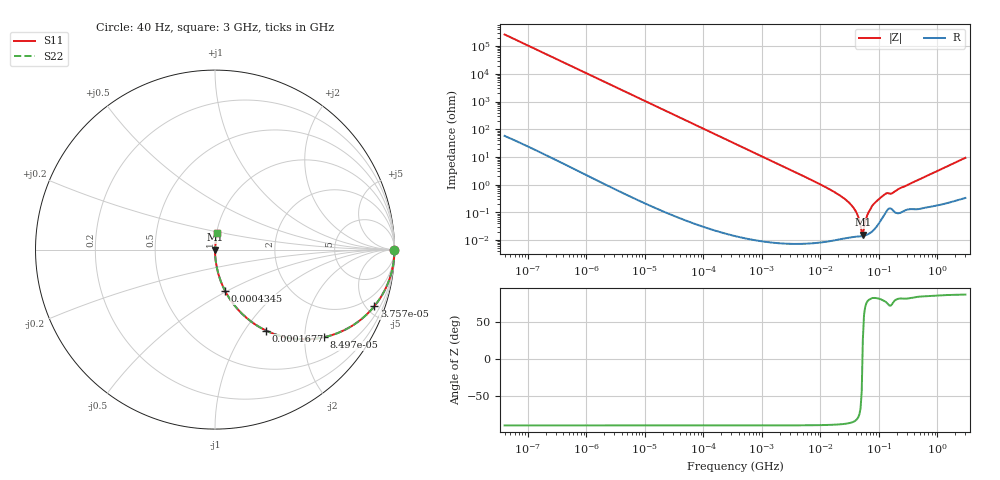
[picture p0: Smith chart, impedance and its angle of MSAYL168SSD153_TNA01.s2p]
! MSAYL168SSD153_TNA01  S-PARAMETER MODEL  ( General Type )
! Model Generated by TAIYO YUDEN Corporation (http://www.ty-top.com)
! Version 3.0
! TAIYO YUDEN Control No. 160201
! Copyright(c) 2003 TAIYO YUDEN CO.,LTD. All Rights Reserved.
! Product Description (link to TY-COMPAS)
! https://ds.yuden.co.jp/TYCOMPAS/or/detail?pn=MSAYL168SSD153KTNA01&u=M
! Products Name : Multilayer Ceramic Capacitors
! Characteristics :
!  Capacitance : 0.015 uF , Rated Voltage : 10V
!  Case Size : 1.6 x 0.8 / 0.063 x 0.031 [mm/inch] , Thickness : 0.8 / 0.031 [mm/inch]
!  (Conditions: Temperature = 25 degC , DC Bias Current/Voltage = 0A / 0V)
! External Node Assignments :
!  1  o---| |---o  2
! GND o---------o GND
! Frequency Range : 0.00004MHz  -  3000MHz  [ 401 STEP ]
# MHz S RI R 50
! Freq[MHz].  S11 Real  S11 Imag  S21 Real  S21 Imag  S12 Real  S12 Imag  S22 Real  S22 Imag
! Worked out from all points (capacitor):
!   401 points, 40 Hz to 3 GHz, reference 50 ohm
!   read as one part in series: C = 15.1 nF near 44 Hz
!   lowest |Z| = 15.8 mohm at 53.08 MHz (marker M1)
!   series resonance near 52.25 MHz, so ESL is about 620 pH
!   S11 on the Smith chart (normalised r, x): 40 Hz: open; 37.58 kHz: 1.00, -5.62; 84.97 kHz: 1.00, -2.49; 167.7 kHz: 1.00, -1.26; 434.5 kHz: 1.00, -0.49; 3 GHz: 1.01, +0.19
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4e-05  1 -0.000379  2.26e-07 0.000379  2.26e-07 0.000379  1 -0.000379
0.000834  0.9999 -0.00789  6.4e-05 0.00789  6.4e-05 0.00789  0.9999 -0.00789
0.017386  0.9736 -0.1602  0.0264 0.1602  0.0264 0.1602  0.9736 -0.1602
0.037575  0.8876 -0.3157  0.1124 0.3157  0.1124 0.3157  0.8876 -0.3157
0.084972  0.6072 -0.4882  0.3928 0.4882  0.3928 0.4882  0.6072 -0.4882
0.167721  0.2841 -0.4508  0.7159 0.4508  0.7159 0.4508  0.2841 -0.4508
0.362475  0.0784 -0.2686  0.9216 0.2686  0.9216 0.2686  0.0784 -0.2686
0.434539  0.0559 -0.2295  0.9441 0.2295  0.9441 0.2295  0.0559 -0.2295
1.349647  0.00616 -0.0777  0.9938 0.0777  0.9938 0.0777  0.00616 -0.0777
7.222098  0.000282 -0.0143  0.9997 0.0143  0.9997 0.0143  0.000282 -0.0143
17.88201  0.000127 -0.00522  0.9999 0.00522  0.9999 0.00522  0.000127 -0.00522
29.4429  0.000127 -0.00246  0.9999 0.00246  0.9999 0.00246  0.000127 -0.00246
38.64618  0.000133 -0.00125  0.9999 0.00125  0.9999 0.00125  0.000133 -0.00125
44.27611  0.000135 -0.000684  0.9999 0.000684  0.9999 0.000684  0.000135 -0.000684
48.47801  0.000137 -0.000315  0.9999 0.000315  0.9999 0.000315  0.000137 -0.000315
53.07868  0.00014 7.23e-05  0.9999 -7.23e-05  0.9999 -7.23e-05  0.00014 7.23e-05
55.54024  0.000144 0.00025  0.9999 -0.00025  0.9999 -0.00025  0.000144 0.00025
66.58224  0.000168 0.001  0.9998 -0.001  0.9998 -0.001  0.000168 0.001
79.8195  0.000227 0.00191  0.9998 -0.00191  0.9998 -0.00191  0.000227 0.00191
120.0322  0.000763 0.00409  0.9992 -0.00409  0.9992 -0.00409  0.000763 0.00409
150.5692  0.00142 0.00456  0.9986 -0.00456  0.9986 -0.00456  0.00142 0.00456
3000  0.0119 0.0921  0.9881 -0.0921  0.9881 -0.0921  0.0119 0.0921
